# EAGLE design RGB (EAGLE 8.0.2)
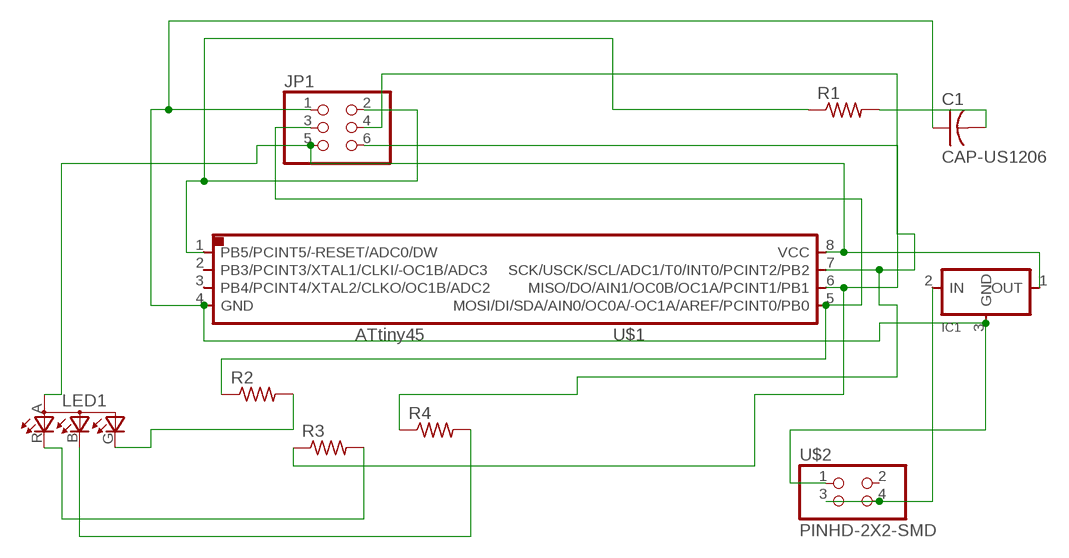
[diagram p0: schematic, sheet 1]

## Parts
C1  CAP-US1206  [C1206]
IC1  REGULATORSOT23  [SOT23]
JP1  PINHD-2X3-SMD  [2X03SMD]
LED1  LEDRGBOLD  [P-LCC-4-3]
R1  RES-US1206  [R1206]
R2  RES-US1206  [R1206]
R3  RES-US1206  [R1206]
R4  RES-US1206  [R1206]
U$1  ATTINY45SI  [SOIC8]
U$2  PINHD-2X2-SMD  [2X02SMD]

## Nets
N$1: C1.1 IC1.3(GND) JP1.1 U$1.4(GND) U$2.1
N$2: JP1.2 R1.1 U$1.1(PB5/PCINT5/-RESET/ADC0/DW)
N$3: JP1.3 R2.1 U$1.5(MOSI/DI/SDA/AIN0/OC0A/-OC1A/AREF/PCINT0/PB0)
N$4: IC1.1(OUT) JP1.5 LED1.A(A2) U$1.8(VCC)
N$5: JP1.6 R3.1 U$1.6(MISO/DO/AIN1/OC0B/OC1A/PCINT1/PB1)
N$6: C1.2 R1.2
N$7: JP1.4 R4.1 U$1.7(SCK/USCK/SCL/ADC1/T0/INT0/PCINT2/PB2)
N$8: IC1.2(IN) U$2.3 U$2.4
N$9: LED1.G(CGREEN) R2.2
N$11: LED1.R(CRED) R3.2
N$13: LED1.B(CBLUE) R4.2
Unconnected: U$1.2(PB3/PCINT3/XTAL1/CLKI/-OC1B/ADC3) U$1.3(PB4/PCINT4/XTAL2/CLKO/OC1B/ADC2) U$2.2

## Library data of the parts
C1 = fab:CAP-US
IC1 = fab:REGULATOR
JP1 = fab:PINHD-2X3-SMD: PIN HEADER
LED1 = fab:LEDRGBOLD: OSRAM Hyper Multi TOPLED® Hyper-Bright LED LATB T686 Source: http://www.osram.convergy.de/
R1-R4 = fab:RES-US: Resistor (US Symbol)
U$1 = fab:ATTINY45
U$2 = fab:PINHD-2X2-SMD

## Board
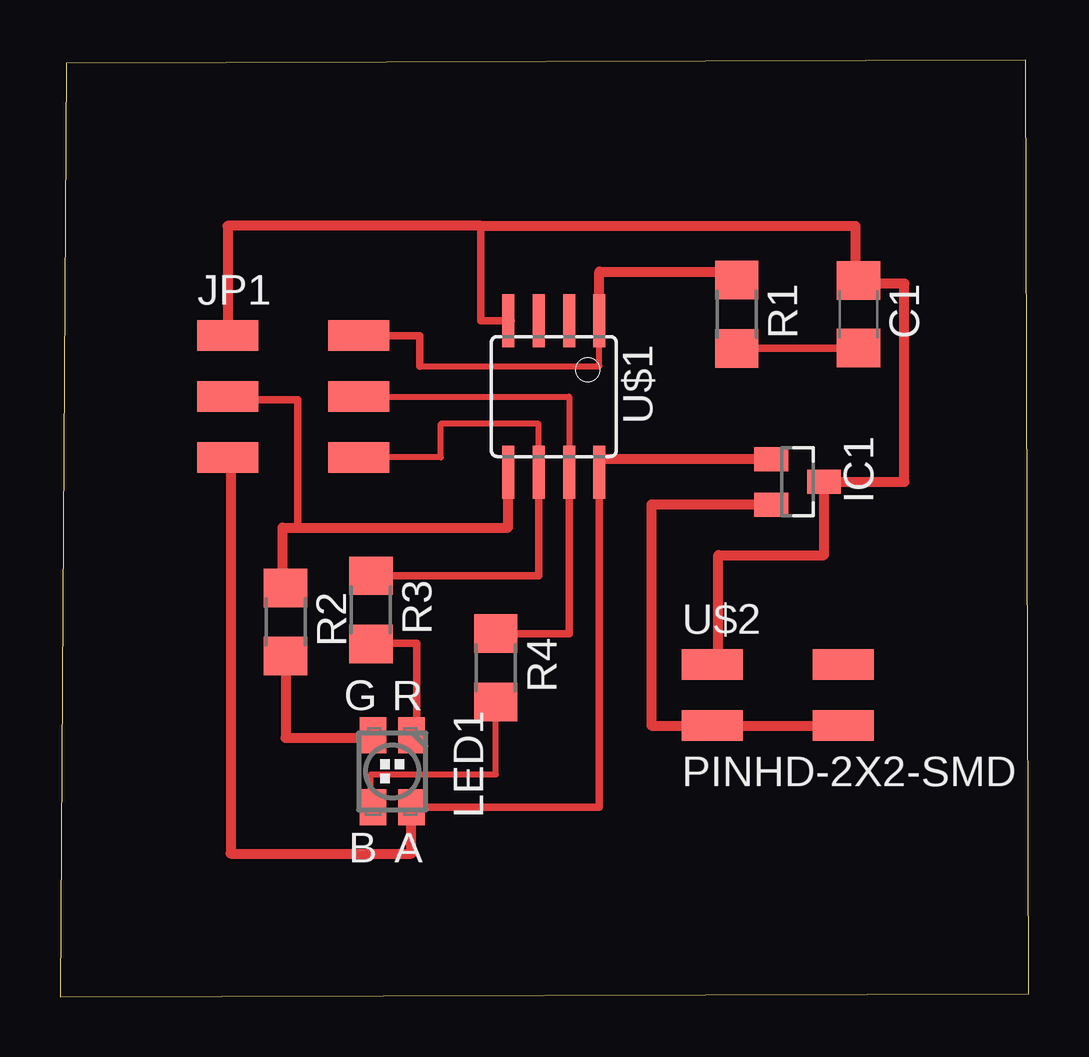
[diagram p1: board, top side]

Size 40.37 x 39.04 mm. Coordinates in mm from the lower left corner, seen from the top.
Outline: 0,0 40.37,0.13 40.24,39.04 0.25,38.91 0,0
Copper layers (1*16): Top 0.035mm / dielectric 1.5mm / Bottom 0.035mm
Design rules "default": minimum track width 10mil, minimum drill 24mil, track to track 8mil, track to pad 8mil, pad to pad 8mil, via to via 8mil, smd to smd 8mil, copper to edge 40mil, drill to drill 8mil, minimum pad ring 10mil, minimum via ring 8mil, stop-mask expansion 4mil, vias tented up to drill 0mil, thermal gap 10mil

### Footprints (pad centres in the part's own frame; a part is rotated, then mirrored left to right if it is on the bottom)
C1206 = smd 1.6 x 1.8: 1 -1.4,0; 2 1.4,0
SOT23 = smd 1 x 1.4: 1 -0.95,-1.1; 2 0.95,-1.1; 3 0,1.1
2X03SMD = smd 2.54 x 1.27: 1 -2.54,2.54; 2 2.92,2.54; 3 -2.54,0; 4 2.92,0; 5 -2.54,-2.54; 6 2.92,-2.54
P-LCC-4-3 = smd 1.1 x 1.5: A -0.8,1.5; B 0.8,1.5; G 0.8,-1.5; R -0.8,-1.5
R1206 = smd 1.6 x 1.803: 1 -1.422,0; 2 1.422,0
SOIC8 = smd 0.5 x 2.2: 1 -1.905,-3.154; 2 -0.645,-3.154; 3 0.625,-3.154; 4 1.895,-3.154; 5 1.905,3.154; 6 0.635,3.154; 7 -0.635,3.154; 8 -1.905,3.154
2X02SMD = smd 2.54 x 1.27: 1 -2.54,1.27; 2 2.92,1.27; 3 -2.54,-1.27; 4 2.92,-1.27

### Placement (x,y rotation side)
C1  33.27,28.45 270 top
IC1  30.73,21.46 270 top
JP1  9.52,25.02 0 top
LED1  13.84,9.4 180 top
R1  28.19,28.45 270 top
R2  9.4,15.62 270 top
R3  12.95,16.13 270 top
R4  18.16,13.72 270 top
U$1  20.57,25.02 180 top
U$2  29.72,12.57 0 top

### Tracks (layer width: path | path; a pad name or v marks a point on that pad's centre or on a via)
N$1
  Top 0.254: 18.67,27.56 U$1.4 18.67,28.19
  Top 0.305: 18.8,28.17 U$1.4 17.53,28.17 17.53,32.13 | C1.1 33.15,29.85 | C1.1 | 33.27,29.72 C1.1 | U$2.1 27.43,13.84
  Top 0.406: 33.15,29.85 33.15,32.13 17.53,32.13 6.98,32.13 JP1.1 | 33.27,29.72 35.18,29.72 35.18,21.46 IC1.3 31.83,18.41 27.43,18.41 27.43,13.84
N$2
  Top 0.254: 14.99,26.29 22.48,26.29 U$1.1
  Top 0.305: JP1.2 14.99,27.56 14.99,26.29 | 28.19,30.23 R1.1
  Top 0.406: U$1.1 22.48,30.23 28.19,30.23
N$3
  Top 0.254: U$1.5 18.67,22.48
  Top 0.305: 6.98,24.77 JP1.3 6.98,24.89 9.91,24.89 9.91,19.56 | R2.1 9.27,17.04
  Top 0.406: U$1.5 18.67,19.56 9.91,19.56 9.27,19.56 9.27,17.04
N$4
  Top 0.305: U$1.8 22.48,22.29 | U$1.8 22.48,7.9 LED1.A 14.6,7.9 | 22.48,22.41 U$1.8
  Top 0.406: IC1.1 22.48,22.41 | JP1.5 7.11,22.48 7.11,5.97 14.64,5.97 LED1.A
N$5
  Top 0.254: JP1.6 15.87,22.48 15.87,23.88 19.94,23.88 U$1.6
  Top 0.305: JP1.6 12.95,22.48 | R3.1 19.94,17.55 U$1.6
N$6
  Top 0.305: R1.2 33.27,27.03 C1.2
N$7
  Top 0.254: 21.21,22.48 U$1.7 21.21,25.02 JP1.4
  Top 0.305: R4.1 21.21,15.14 U$1.7
N$8
  Top 0.305: U$2.4 33.02,11.3 | 24.64,20.19 24.64,20.39
  Top 0.406: U$2.4 U$2.3 24.64,11.3 24.64,20.19 24.64,20.51 IC1.2
N$9
  Top 0.305: 13.04,10.79 LED1.G
  Top 0.406: R2.2 9.4,10.79 13.04,10.79
N$11
  Top 0.305: LED1.R 14.86,10.9 14.86,14.73 12.95,14.73 R3.2
N$13
  Top 0.254: 12.95,7.9 12.95,9.27 18.16,9.27 R4.2
  Top 0.305: LED1.B 12.95,7.9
